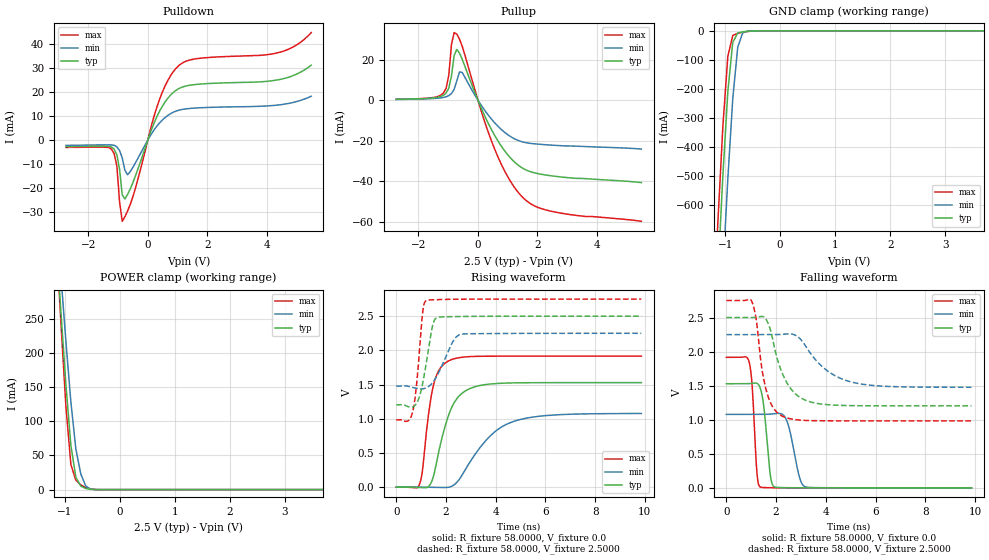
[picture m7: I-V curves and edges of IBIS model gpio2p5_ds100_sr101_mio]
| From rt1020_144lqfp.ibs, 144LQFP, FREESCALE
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[Model] gpio2p5_ds100_sr101_mio
|   Model gpio2p5_ds100_sr101_mio
| This model was characterised for following simulation conditions:
| External (pad) voltage:
|   - Typ: 2.5V,   - Min: 2.25V,   - Max: 2.75V
| Library cells for typ/min/max conditions are connected as defined below:
|  pad - External Pad
|  ipp_do - Core Input
|  ipp_obe - Output Buffer Enable
|  esd_boost - ovdd
|  ipp_dse0 - vssi
|  ipp_dse1 - vssi
|  ipp_dse2 - vddi
|  ipp_fsel0 - vddi
|  ipp_fsel1 - vssi
|  ipp_ina - ipp_ina
|  ipp_ind - ipp_ind
|  ipp_pwr_stable - vddi
|  ipp_sre - vddi
|  ovdd - ovdd
|  ovss - ovss
|  vddi - vddi
|  vssi - vssi
| All other pins connected to ground
Model_type I/O
Polarity   Non-Inverting
Enable   Active-High
Vinl =   0.7500V
Vinh =   1.7500V
Vmeas =  1.2500V
Cref =   0.0F
Rref =   58.0000
Vref =   1.2500V
C_comp   1.2356pF   1.1994pF   1.2834pF
|C_comp_pullup   0.6221pF   0.6388pF   0.6072pF
|C_comp_pulldown   0.5474pF   0.5787pF   0.5258pF
[Model Spec]
| variable   typ   min   max
Vinh   1.7500V   1.5750V   1.9250V
Vinl   0.7500V   0.6750V   0.8250V
S_overshoot_high   2.5000V   2.2500V   2.7500V
S_overshoot_low   0.0V   0.0V   0.0V
Vmeas   1.2500V   1.1250V   1.3750V
Vref   1.2500V   1.1250V   1.3750V
Cref   0.0F   0.0F   0.0F
Rref   58.0000   58.0000   58.0000
[Temperature Range]   25.0000   0.1050k   -20.0000
[Voltage Range]   2.5000V   2.2500V   2.7500V
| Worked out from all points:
|   slope of the pulldown table from 0 to 0.375 V, typ, clamps not added: 32.5 ohm
|   slope of the pullup table from 0 to 0.375 V, typ, clamps not added: 30.7 ohm
|   GND clamp passes 1 mA (typ) near -0.54 V on its own axis
|   POWER clamp passes 1 mA (typ) near -0.57 V on its own axis
|   rising waveform, R_fixture 58.0000, V_fixture 0.0: 20-80 % time 721ps typ, 1.45ns min, 429ps max; typ from 0 V to 1.53 V
|   rising waveform, R_fixture 58.0000, V_fixture 2.5000: 20-80 % time 363ps typ, 586ps min, 251ps max; typ from 1.2 V to 2.5 V
|   falling waveform, R_fixture 58.0000, V_fixture 0.0: 20-80 % time 233ps typ, 362ps min, 169ps max; typ from 1.53 V to 0 V
|   falling waveform, R_fixture 58.0000, V_fixture 2.5000: 20-80 % time 747ps typ, 1.28ns min, 453ps max; typ from 2.5 V to 1.2 V
[Pulldown]
|Voltage   I(typ)   I(min)   I(max)
-2.75V    -2.761mA   -2.233mA   -3.086mA
-1.22V    -2.901mA   -2.018mA   -3.8mA
-1.04V    -6.257mA   -2.877mA   -11.05mA
-950mV    -12.24mA   -4.387mA   -25.89mA
-860mV    -22.93mA   -7.491mA   -33.98mA
-680mV    -22.73mA   -14.5mA    -29.66mA
-410mV    -14.8mA    -9.393mA   -19.86mA
400mV     12.16mA    7.219mA    17.16mA
1.03V     21.43mA    12.43mA    31mA
1.66V     23.3mA     13.44mA    34.06mA
4.36V     25.14mA    14.62mA    36.46mA
5.5V      31.32mA    18.34mA    44.95mA
[Pullup]
|Voltage   I(typ)   I(min)   I(max)
-2.75V    410uA      350uA      450uA
-1.16V    2.417mA    1.339mA    3.554mA
-980mV    5.918mA    2.226mA    12.31mA
-890mV    11.95mA    3.26mA     27.43mA
-800mV    21.99mA    5.348mA    33.28mA
-710mV    24.98mA    9.532mA    32.5mA
-530mV    20.16mA    13.63mA    26.57mA
550mV     -17.02mA   -10.92mA   -23.61mA
1V        -26.84mA   -16.97mA   -37.61mA
1.54V     -33.79mA   -20.71mA   -48.33mA
2.62V     -37.53mA   -22.28mA   -55.18mA
5.5V      -40.6mA    -24.07mA   -59.65mA
[GND_clamp]
|Voltage   I(typ)   I(min)   I(max)
-2.75V    -7.488A    -7.708A    -7.379A
-1.22V    -1.193A    -1.537A    -1.012A
-1.13V    -835.6mA   -1.18A     -654.7mA
-1.04V    -497.8mA   -833mA     -328mA
-950mV    -208.9mA   -508.7mA   -87.54mA
-860mV    -39.89mA   -232.5mA   -15.89mA
-770mV    -7.264mA   -56.44mA   -8.363mA
-680mV    -3.422mA   -7.048mA   -4.851mA
-590mV    -1.552mA   -1.455mA   -2.251mA
-500mV    -482.7uA   -438.2uA   -698.4uA
5.5V      0A         0A         0A
[POWER_clamp]
|Voltage   I(typ)   I(min)   I(max)
-2.75V    2.386A     2.288A     2.687A
-1.16V    368.2mA    410.8mA    372.9mA
-1.07V    258.5mA    311.8mA    242.5mA
-980mV    153.1mA    216.2mA    121.1mA
-890mV    64.5mA     128mA      36.56mA
-800mV    18.16mA    59.6mA     13.82mA
-710mV    5.012mA    22.76mA    6.935mA
-620mV    1.706mA    5.315mA    2.959mA
-530mV    383.1uA    636.8uA    795.1uA
-440mV    42.36uA    66.97uA    84.45uA
5.5V      0A         0A         0A
[Ramp]
| variable   typ   min   max
dV/dt_r  0.9172/0.7212n   0.6465/1.4501n   1.1497/0.4291n
dV/dt_f  0.7773/0.7468n   0.4638/1.2851n   1.0598/0.4532n
R_load = 58.0000
[Rising Waveform]
R_fixture= 58.0000
V_fixture= 0.0
V_fixture_min= 0.0
V_fixture_max= 0.0
|time   V(typ)   V(min)   V(max)
0s        1.003nV    3.879nV    3.167nV
938.3ps   -4.882mV   140uV      42.29mV
1.05ns    -6.753mV   -251.8uV   224.8mV
1.276ns   1.823mV    -1.416mV   999mV
1.489ns   146.8mV    -3.022mV   1.477V
2.073ns   1.015V     -3.552mV   1.84V
2.87ns    1.426V     311.2mV    1.907V
3.769ns   1.508V     744.7mV    1.916V
4.664ns   1.525V     953.7mV    1.916V
9.86ns    1.529V     1.077V     1.916V
[Rising Waveform]
R_fixture= 58.0000
V_fixture= 2.5000
V_fixture_min= 2.2500
V_fixture_max= 2.7500
|time   V(typ)   V(min)   V(max)
0s        1.204V     1.477V     983.7mV
466.8ps   1.179V     1.477V     967.4mV
663.4ps   1.172V     1.458V     1.103V
822.5ps   1.228V     1.444V     1.511V
1.062ns   1.514V     1.438V     2.552V
1.213ns   1.823V     1.453V     2.729V
1.558ns   2.456V     1.578V     2.742V
2.271ns   2.494V     2.124V     2.748V
2.595ns   2.496V     2.235V     2.749V
9.86ns    2.5V       2.25V      2.75V
[Falling Waveform]
R_fixture= 58.0000
V_fixture= 0.0
V_fixture_min= 0.0
V_fixture_max= 0.0
|time   V(typ)   V(min)   V(max)
0s        1.529V     1.078V     1.916V
920ps     1.53V      1.078V     1.844V
1.047ns   1.535V     1.078V     1.449V
1.23ns    1.535V     1.078V     223.6mV
1.365ns   1.462V     1.078V     12.79mV
1.768ns   192.4mV    1.083V     2.332mV
1.942ns   13.46mV    1.089V     1.553mV
2.442ns   2.357mV    976.2mV    485.2uV
3.168ns   692uV      17.26mV    88.33uV
9.86ns    157.2nV    1.712uV    -295.7nV
[Falling Waveform]
R_fixture= 58.0000
V_fixture= 2.5000
V_fixture_min= 2.2500
V_fixture_max= 2.7500
|time   V(typ)   V(min)   V(max)
0s        2.5V       2.25V      2.75V
1.025ns   2.499V     2.25V      2.736V
1.185ns   2.502V     2.25V      2.51V
1.414ns   2.517V     2.25V      1.788V
1.612ns   2.466V     2.25V      1.423V
2.283ns   1.655V     2.255V     1.047V
3.168ns   1.288V     2.094V     990.6mV
3.917ns   1.226V     1.76V      984.7mV
4.981ns   1.208V     1.558V     983.7mV
9.86ns    1.204V     1.477V     983.7mV
